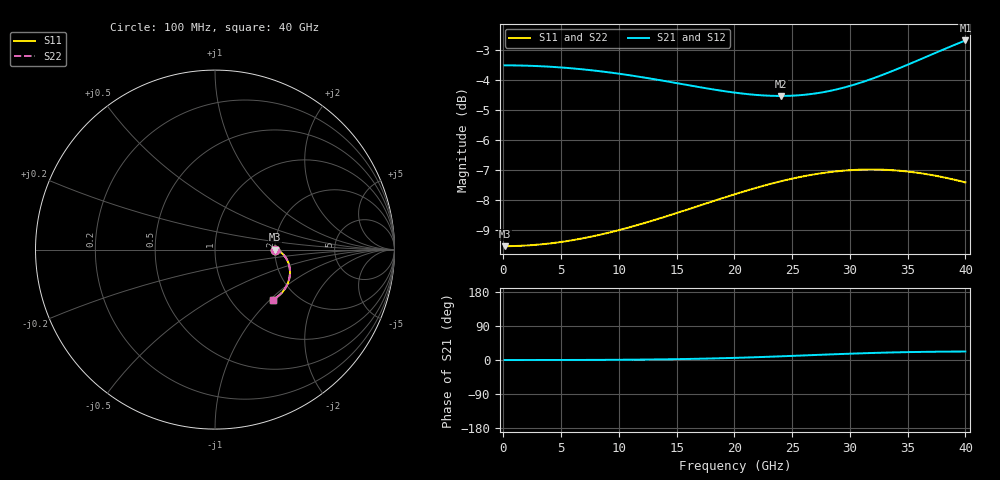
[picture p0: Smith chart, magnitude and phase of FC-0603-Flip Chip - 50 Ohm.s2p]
!Vishay Thin-Film
!FC Family
!Case Size 0603
!Assembly Style Flip Chip
!11/9/2015
!thinfilm@vishay.com
# GHz S MA R 50
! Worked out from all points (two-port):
!   101 points, 100 MHz to 40 GHz, reference 50 ohm
!   highest |S21| = -2.69 dB at 40 GHz (marker M1); lowest = -4.5 dB at 24.04 GHz (marker M2)
!   |S21| within 3 dB of the highest: start of sweep to end of sweep
!   lowest |S11| = -9.5 dB at 100 MHz (marker M3), VSWR 2.00, Z = 100 - j1.55e-06 ohm
!   |S11| at or under -10 dB: nowhere
!   |S22| runs from -9.5 to -7.0 dB; largest |S21 - S12| = 0
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0.1  0.3333 -0.0  0.6667 0.0  0.6667 0.0  0.3333 -0.0
3.292  0.3357 -0.0  0.6643 0.0  0.6643 0.0  0.3357 -0.0
4.888  0.3385 -0.1  0.6615 0.1  0.6615 0.1  0.3385 -0.1
6.883  0.3436 -0.4  0.6565 0.2  0.6565 0.2  0.3436 -0.4
10.474  0.3565 -1.3  0.6437 0.7  0.6437 0.7  0.3565 -1.3
13.666  0.3715 -2.8  0.6293 1.7  0.6293 1.7  0.3715 -2.8
15.262  0.3799 -3.9  0.6215 2.4  0.6215 2.4  0.3799 -3.9
16.858  0.3887 -5.2  0.6138 3.3  0.6138 3.3  0.3887 -5.2
18.454  0.3978 -6.7  0.6067 4.4  0.6067 4.4  0.3978 -6.7
20.05  0.4068 -8.4  0.6004 5.7  0.6004 5.7  0.4068 -8.4
22.045  0.4177 -10.8  0.5949 7.6  0.5949 7.6  0.4177 -10.8
24.04  0.4276 -13.6  0.5929 9.7  0.5929 9.7  0.4276 -13.6
25.636  0.4344 -16.0  0.5945 11.6  0.5945 11.6  0.4344 -16.0
26.833  0.4387 -17.9  0.5979 13.0  0.5979 13.0  0.4387 -17.9
28.429  0.4432 -20.6  0.6054 14.9  0.6054 14.9  0.4432 -20.6
30.025  0.4461 -23.3  0.6163 16.7  0.6163 16.7  0.4461 -23.3
31.621  0.4472 -26.2  0.6304 18.2  0.6304 18.2  0.4472 -26.2
33.616  0.4461 -29.8  0.6517 19.9  0.6517 19.9  0.4461 -29.8
35.212  0.4432 -32.7  0.6709 20.9  0.6709 20.9  0.4432 -32.7
36.808  0.4388 -35.5  0.6914 21.6  0.6914 21.6  0.4388 -35.5
38.404  0.4328 -38.2  0.7124 22.1  0.7124 22.1  0.4328 -38.2
40  0.4256 -40.9  0.7334 22.3  0.7334 22.3  0.4256 -40.9
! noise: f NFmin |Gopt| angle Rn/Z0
0.1  9.643e-16  1  1.333e-21  1
4.489  9.334e-08  1  -1.354e-15  1.02
8.878  9.859e-08  1  2.457e-15  1.077
13.27  2.893e-15  1  0  1.168
17.66  -1.446e-15  1  -2.521e-15  1.271
22.05  -2.893e-15  1  -8.43e-16  1.333
26.43  6.75e-15  1  8.78e-16  1.272
30.82  -4.822e-16  1  3.858e-15  1.062
35.21  -9.643e-16  1  -6.75e-15  0.7851
40  1.929e-15  1  -1.207e-06  0.5223
